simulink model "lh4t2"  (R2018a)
settings: Solver=ode45  StartTime=0.0  StopTime=40.0  RelTol=1e-3  AbsTol=1e-6
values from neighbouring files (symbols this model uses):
  Aa = [ -R/L,     0, -k1/L,    0, 0    [lh4t2_m.m]
  Ab = [ -R/L, 0, -k1/L    [lh4t2_m.m]
  Ac = [0,                     1    [lh4t2_m.m]
  Ba = [1/L    [lh4t2_m.m]
  Bb = [1/L    [lh4t2_m.m]
  Bc = [        0    [lh4t2_m.m]

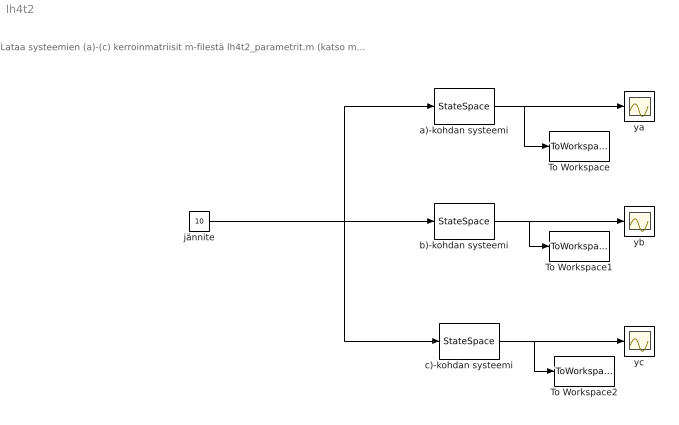
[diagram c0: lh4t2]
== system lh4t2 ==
  note: Lataa systeemien (a)-(c) kerroinmatriisit m-filestä lh4t2_parametrit.m (katso mitä se on syönyt sisäänsä)
  To Workspace : ToWorkspace  VariableName=ya  SampleTime=-1
  To Workspace1 : ToWorkspace  VariableName=yb  SampleTime=-1
  To Workspace2 : ToWorkspace  VariableName=yc  SampleTime=-1
  a)-kohdan systeemi : StateSpace  A=Aa  B=Ba  C=[0 0 0 0 1]  D=0  InitialCondition=[0;0;0;0;0]
  b)-kohdan systeemi : StateSpace  A=Ab  B=Bb  C=[0 0 1]  D=0  InitialCondition=[0;0;0]
  c)-kohdan systeemi : StateSpace  A=Ac  B=Bc  C=[0 1]  D=0  InitialCondition=[0;0]
  jännite : Constant  Value=10
  ya : Scope
  yb : Scope
  yc : Scope
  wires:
  a)-kohdan systeemi/1 -> To Workspace/1, ya/1
  c)-kohdan systeemi/1 -> To Workspace2/1, yc/1
  b)-kohdan systeemi/1 -> To Workspace1/1, yb/1
  jännite/1 -> c)-kohdan systeemi/1, b)-kohdan systeemi/1, a)-kohdan systeemi/1
